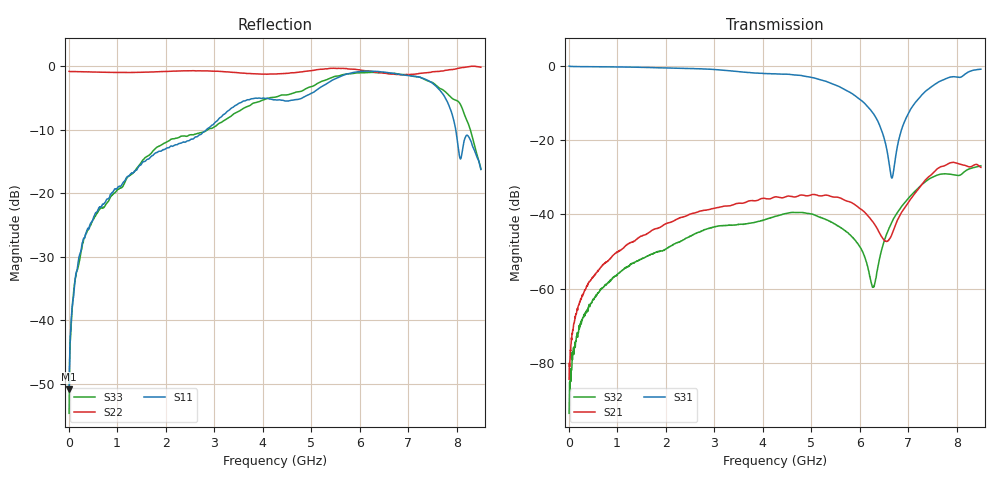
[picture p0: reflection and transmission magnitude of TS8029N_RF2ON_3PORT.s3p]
!Created with skrf (http://scikit-rf.org).
# GHz S RI R 50.0
!freq ReS11 ImS11 ReS12 ImS12 ReS13 ImS13
! ReS21 ImS21 ReS22 ImS22 ReS23 ImS23
! ReS31 ImS31 ReS32 ImS32 ReS33 ImS33
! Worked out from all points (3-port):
!   1601 points, 10 MHz to 8.5 GHz, reference 50 ohm
!   strongest paths, dB at 10 MHz, 2.132 GHz, 4.255 GHz, 6.378 GHz, 8.5 GHz:
!     S31: 0.0, -0.6, -2.1, -14.9, -0.9
!     S21: -84.4, -42.0, -35.3, -44.2, -27.3
!     S32: -93.6, -48.3, -40.5, -54.1, -26.9
!   lowest |S11| = -50.8 dB at 10 MHz (marker M1), VSWR 1.01, Z = 50 + j0.286 ohm
!   |S11| at or under -10 dB: start of sweep to 2.845 GHz; 7.981 GHz to end of sweep
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0.01  0.000318 0.00286  2.1e-05 6.77e-05  0.9947 -0.00838
      4.31e-05 4.19e-05  -0.9055 0.0035  1.55e-05 1.47e-05
      0.9947 -0.00824  4.48e-06 2.05e-05  0.00166 0.000849
0.1426563  0.00861 -0.0203  7.57e-05 0.000416  0.9812 -0.0554
           8.56e-05 0.000422  -0.9016 0.0344  6.02e-05 -0.000198
           0.9813 -0.0554  6.48e-05 -0.000177  0.00665 -0.0207
0.6149125  -0.00305 -0.0755  -0.000118 0.00176  0.95 -0.2236
           -0.000127 0.00176  -0.8802 0.153  -0.000513 -0.000701
           0.9502 -0.2235  -0.000503 -0.000731  -0.01 -0.0724
4.255  -0.5407 0.034  0.00885 0.0148  -0.0802 -0.7815
       0.00877 0.0148  -0.3159 0.804  -0.000288 0.00936
       -0.0813 -0.7799  -0.000248 0.00941  -0.5673 -0.00795
5.666462  -0.5438 0.6478  0.0138 0.00786  -0.3571 -0.3375
          0.0138 0.00785  -0.00719 0.9548  0.00466 0.00421
          -0.3574 -0.3375  0.00467 0.0042  -0.5417 0.6613
6.276681  -0.2254 0.8806  0.00695 0.00376  -0.2105 -0.0958
          0.00693 0.00374  0.0297 0.9009  -0.000254 0.00102
          -0.2107 -0.0959  -0.000207 0.00103  -0.3762 0.8067
6.664038  0.0344 0.8755  -0.00113 0.00524  -0.00382 -0.0307
          -0.00116 0.00524  0.1553 0.8486  -0.00748 0.00242
          -0.00391 -0.0306  -0.00746 0.00238  0.0833 0.8698
7.173438  0.4609 0.6829  -0.00799 0.0189  0.2375 -0.2397
          -0.00806 0.0189  0.3813 0.7769  -0.0136 0.0168
          0.2377 -0.2398  -0.0135 0.0167  0.5827 0.5797
7.926925  0.3909 0.0107  0.0207 0.046  0.0443 -0.7162
          0.0208 0.046  0.5653 0.7485  0.00951 0.0331
          0.0437 -0.7163  0.00941 0.033  0.4889 0.2495
8.5  0.092 0.1229  0.0241 0.0357  -0.2546 -0.8689
     0.0242 0.0357  0.5286 0.821  0.0186 0.0413
     -0.2553 -0.8684  0.0185 0.0413  0.1542 -0.0115
